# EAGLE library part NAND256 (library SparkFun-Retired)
NAND flash Not in catalog
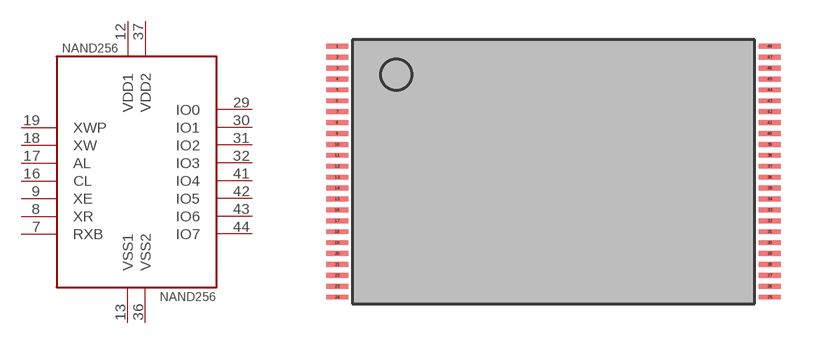
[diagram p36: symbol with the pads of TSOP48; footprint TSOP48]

Designator prefix -

## NAND256  [TSOP48]
7  RXB
8  XR
9  XE
12  VDD1
13  VSS1
16  CL
17  AL
18  XW
19  XWP
29  IO0
30  IO1
31  IO2
32  IO3
36  VSS2
37  VDD2
41  IO4
42  IO5
43  IO6
44  IO7

## Footprint TSOP48 (pad centres in mm)
smd 1 x 0.22: 1 -0.7,11.8; 2 -0.7,11.3; 3 -0.7,10.8; 4 -0.7,10.3; 5 -0.7,9.8; 6 -0.7,9.3; 7 -0.7,8.8; 8 -0.7,8.3; 9 -0.7,7.8; 10 -0.7,7.3; 11 -0.7,6.8; 12 -0.7,6.3; 13 -0.7,5.8; 14 -0.7,5.3; 15 -0.7,4.8; 16 -0.7,4.3; 17 -0.7,3.8; 18 -0.7,3.3; 19 -0.7,2.8; 20 -0.7,2.3; 21 -0.7,1.8; 22 -0.7,1.3; 23 -0.7,0.8; 24 -0.7,0.3; 25 19.1,0.3; 26 19.1,0.8; 27 19.1,1.3; 28 19.1,1.8; 29 19.1,2.3; 30 19.1,2.8; 31 19.1,3.3; 32 19.1,3.8; 33 19.1,4.3; 34 19.1,4.8; 35 19.1,5.3; 36 19.1,5.8; 37 19.1,6.3; 38 19.1,6.8; 39 19.1,7.3; 40 19.1,7.8; 41 19.1,8.3; 42 19.1,8.8; 43 19.1,9.3; 44 19.1,9.8; 45 19.1,10.3; 46 19.1,10.8; 47 19.1,11.3; 48 19.1,11.8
